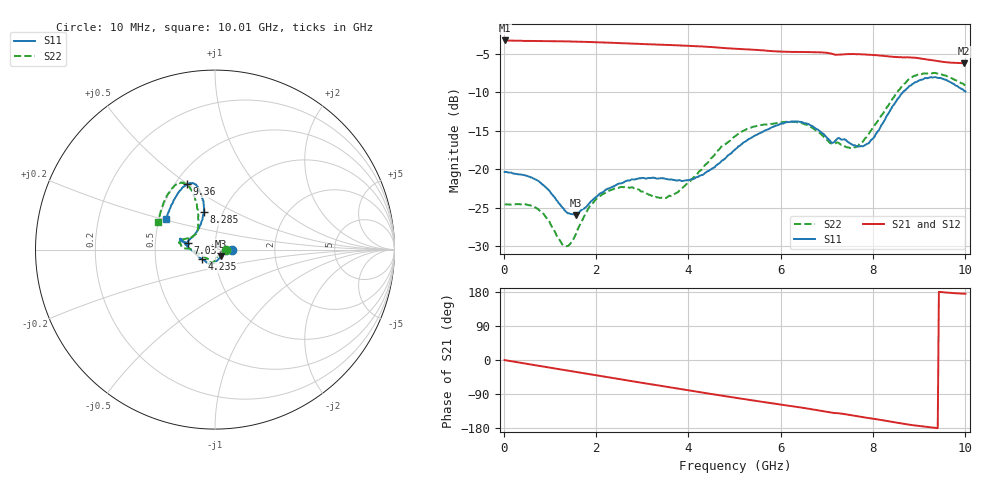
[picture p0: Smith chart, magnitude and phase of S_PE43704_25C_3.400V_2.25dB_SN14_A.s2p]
! Device ID: PE43704
! Dir: z:\PE43704\PE43704_Char_1_20130516\PE43704\AMB\3p400V\2p25dB
! Serial: 14
! Insertion: A
! Impedance: 50 ohm
! Temp: Amb
! VDD: 3.400V
! Attenuation Step: 2.25dB
! IDD: 1.140999e-01mA
#  Hz  S  RI  R  50
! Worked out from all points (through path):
!   401 points, 10 MHz to 10.01 GHz, reference 50 ohm
!   highest |S21| = -3.28 dB at 10 MHz (marker M1); lowest = -6.2 dB at 9.985 GHz (marker M2)
!   group delay of S21, straight-line fit = 52.7 ps
!   lowest |S11| = -25.9 dB at 1.56 GHz (marker M3), VSWR 1.11, Z = 53.3 - j4.09 ohm
!   |S11| at or under -10 dB: start of sweep to 8.654 GHz
!   |S22| runs from -30.0 to -7.5 dB; largest |S21 - S12| = 0.0044
!   S11 on the Smith chart (normalised r, x): 10 MHz: 1.21, +0.00; 4.235 GHz: 0.86, -0.09; 7.035 GHz: 0.73, +0.06; 8.285 GHz: 0.81, +0.35; 9.36 GHz: 0.57, +0.49; 10.01 GHz: 0.55, +0.21
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1e7  0.0961 4.61e-05  0.6858 -0.00287  0.6862 -0.00262  0.0591 0.000284
7.1e8  0.0841 0.0129  0.6586 -0.17  0.6586 -0.1698  0.0527 0.018
1.31e9  0.0508 -0.0192  0.6046 -0.3035  0.6047 -0.3033  0.0287 -0.0138
1.56e9  0.0331 -0.0383  0.5735 -0.3544  0.5734 -0.3544  0.0168 -0.0343
1.685e9  0.0248 -0.0486  0.5559 -0.379  0.5559 -0.3788  0.0102 -0.0448
1.985e9  0.00681 -0.0655  0.5093 -0.4323  0.5093 -0.4322  -0.00155 -0.0636
2.385e9  -0.0113 -0.077  0.44 -0.4937  0.4402 -0.4936  -0.0153 -0.0732
3.36e9  -0.0327 -0.0809  0.2479 -0.5948  0.2485 -0.5945  -0.0326 -0.0567
3.735e9  -0.0457 -0.0712  0.1683 -0.6159  0.169 -0.6157  -0.0543 -0.0443
4.235e9  -0.0732 -0.0535  0.0596 -0.6252  0.0602 -0.6251  -0.0951 -0.0195
5.01e9  -0.1341 1.52e-05  -0.0994 -0.5982  -0.0991 -0.5986  -0.1636 0.00608
5.985e9  -0.1875 0.0593  -0.2642 -0.518  -0.2617 -0.5182  -0.1983 0.0364
6.685e9  -0.1855 0.0462  -0.3718 -0.4405  -0.3723 -0.4399  -0.177 0.057
7.035e9  -0.1529 0.0378  -0.4191 -0.3837  -0.4184 -0.385  -0.1399 0.0605
7.635e9  -0.1194 0.0766  -0.473 -0.2979  -0.4728 -0.2983  -0.0991 0.0979
7.96e9  -0.0869 0.1275  -0.4975 -0.2417  -0.4976 -0.2433  -0.0935 0.1523
8.285e9  -0.0624 0.2075  -0.5102 -0.1828  -0.5097 -0.1848  -0.098 0.2269
8.36e9  -0.0614 0.2275  -0.5127 -0.1679  -0.5121 -0.1696  -0.1007 0.2467
8.835e9  -0.0911 0.339  -0.5255 -0.0791  -0.5223 -0.0807  -0.1543 0.359
9.36e9  -0.1579 0.3639  -0.5067 -0.00633  -0.5073 -0.00485  -0.225 0.3567
9.985e9  -0.2662 0.1828  -0.4865 0.0435  -0.4873 0.0456  -0.3122 0.1649
1.001e10  -0.2711 0.1707  -0.488 0.0446  -0.4898 0.0457  -0.3151 0.1556
